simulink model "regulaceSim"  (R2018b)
settings: Solver=ode5  StartTime=0.0  StopTime=80  FixedStep=0.001  RelTol=1e-3  AbsTol=1e-6
undefined symbols (not defined in the file or in its folder): Crane3D_Center
libraries: simulink x5

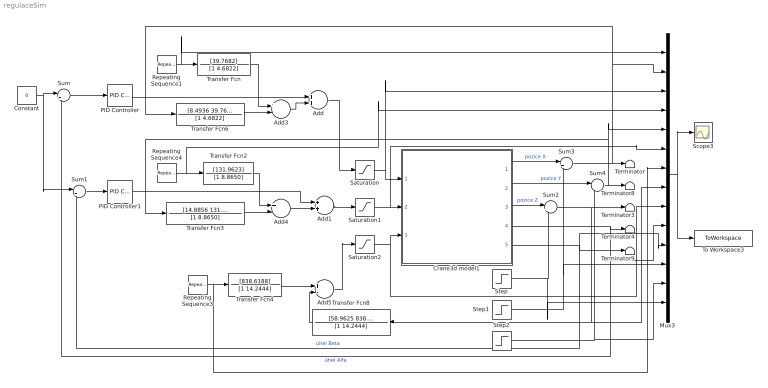
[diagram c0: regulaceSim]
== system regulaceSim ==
  Add : Sum
  Add1 : Sum
  Add3 : Sum  Inputs=+-
  Add4 : Sum  Inputs=+-
  Add5 : Sum  Inputs=+-
  Constant : Constant  Value=0
  Crane3d model1 : Subsystem  mask{RR=off, x0=[0.001, 0, 0.001, 0, 0, 0, 0, 0, 0.001, 0, -1]}
      mask prompts: RR "Model with constant length"; x0 "Initial conditions:[x,x',y,y',alfa,alfa',beta,beta',z,z',t]"
  Mux3 : Mux  Inputs=14
  PID Controller : simulink/Continuous/PID Controller  Controller=P  Form=Parallel  TimeDomain=Continuous-time  SampleTime=-1  IntegratorMethod=Forward Euler  FilterMethod=Forward Euler  ControllerParametersSource=internal  P=-4.5  I=1  D=0  UseFilter=on  N=100  TunerSelectOption=Transfer Function Based (PID Tuner App)  InitialConditionSource=internal  InitialConditionForIntegrator=0  InitialConditionForFilter=0  DifferentiatorICPrevScaledInput=0  ExternalReset=none  TrackingMode=off  Kt=1  LimitOutput=off  UpperSaturationLimit=inf  LowerSaturationLimit=-inf  LinearizeAsGain=on  AntiWindupMode=none  Kb=1  POutMin=[]  POutMax=[]  IOutMin=[]  IOutMax=[]  DOutMin=[]  DOutMax=[]  NOutMin=[]  NOutMax=[]  SumOutMin=[]  SumOutMax=[]  SaturationOutMin=[]  SaturationOutMax=[]  PParamMin=[]  PParamMax=[]  IParamMin=[]  IParamMax=[]  DParamMin=[]  DParamMax=[]  NParamMin=[]  NParamMax=[]  KbParamMin=[]  KbParamMax=[]  KtParamMin=[]  KtParamMax=[]  KbOutMin=[]  KbOutMax=[]  KtOutMin=[]  KtOutMax=[]  IntegratorOutMin=[]  IntegratorOutMax=[]  FilterOutMin=[]  FilterOutMax=[]  SumI1OutMin=[]  SumI1OutMax=[]  SumI2OutMin=[]  SumI2OutMax=[]  SumI3OutMin=[]  SumI3OutMax=[]  SumI4OutMin=[]  SumI4OutMax=[]  SumDOutMin=[]  SumDOutMax=[]  DifferentiatorOutMin=[]  DifferentiatorOutMax=[]  FilterDiffOutCoefMin=[]  FilterDiffOutCoefMax=[]  ReciprocalOutMin=[]  ReciprocalOutMax=[]  SumDenOutMin=[]  SumDenOutMax=[]  SumNumOutMin=[]  SumNumOutMax=[]  DivideOutMin=[]  DivideOutMax=[]  IntegratorContinuousStateAttributes=''  IntegratorStateMustResolveToSignalObject=off  IntegratorRTWStateStorageClass=Auto  FilterContinuousStateAttributes=''  FilterStateMustResolveToSignalObject=off  FilterRTWStateStorageClass=Auto  ParallelPVariant=InternalParameters  IdealPVariant=Disabled  IVariant=Disabled  DVariant=Disabled  IntegratorVariant=Disabled  SatVariant=Disabled  AWVariant=Disabled  PCopyVariant=Disabled  TRVariant=Disabled  FdbkBlocksVariant=Forward  IdealPFdbkVariant=Disabled  SatFdbkVariant=Disabled  DerivativeFilterVariant=Disabled  NVariant=Disabled  NCopyVariant=Disabled_SignalSpec  FilterICVariant=Disabled  IntegratorICVariant=Disabled  ExternalResetVariant=Disabled  TRSumVariant=Passthrough  SumFdbkVariant=Disabled  SumVariant=Passthrough_P
  PID Controller1 : simulink/Continuous/PID Controller  Controller=P  Form=Parallel  TimeDomain=Continuous-time  SampleTime=-1  IntegratorMethod=Forward Euler  FilterMethod=Forward Euler  ControllerParametersSource=internal  P=-4.5  I=1  D=0  UseFilter=on  N=100  TunerSelectOption=Transfer Function Based (PID Tuner App)  InitialConditionSource=internal  InitialConditionForIntegrator=0  InitialConditionForFilter=0  DifferentiatorICPrevScaledInput=0  ExternalReset=none  TrackingMode=off  Kt=1  LimitOutput=off  UpperSaturationLimit=inf  LowerSaturationLimit=-inf  LinearizeAsGain=on  AntiWindupMode=none  Kb=1  POutMin=[]  POutMax=[]  IOutMin=[]  IOutMax=[]  DOutMin=[]  DOutMax=[]  NOutMin=[]  NOutMax=[]  SumOutMin=[]  SumOutMax=[]  SaturationOutMin=[]  SaturationOutMax=[]  PParamMin=[]  PParamMax=[]  IParamMin=[]  IParamMax=[]  DParamMin=[]  DParamMax=[]  NParamMin=[]  NParamMax=[]  KbParamMin=[]  KbParamMax=[]  KtParamMin=[]  KtParamMax=[]  KbOutMin=[]  KbOutMax=[]  KtOutMin=[]  KtOutMax=[]  IntegratorOutMin=[]  IntegratorOutMax=[]  FilterOutMin=[]  FilterOutMax=[]  SumI1OutMin=[]  SumI1OutMax=[]  SumI2OutMin=[]  SumI2OutMax=[]  SumI3OutMin=[]  SumI3OutMax=[]  SumI4OutMin=[]  SumI4OutMax=[]  SumDOutMin=[]  SumDOutMax=[]  DifferentiatorOutMin=[]  DifferentiatorOutMax=[]  FilterDiffOutCoefMin=[]  FilterDiffOutCoefMax=[]  ReciprocalOutMin=[]  ReciprocalOutMax=[]  SumDenOutMin=[]  SumDenOutMax=[]  SumNumOutMin=[]  SumNumOutMax=[]  DivideOutMin=[]  DivideOutMax=[]  IntegratorContinuousStateAttributes=''  IntegratorStateMustResolveToSignalObject=off  IntegratorRTWStateStorageClass=Auto  FilterContinuousStateAttributes=''  FilterStateMustResolveToSignalObject=off  FilterRTWStateStorageClass=Auto  ParallelPVariant=InternalParameters  IdealPVariant=Disabled  IVariant=Disabled  DVariant=Disabled  IntegratorVariant=Disabled  SatVariant=Disabled  AWVariant=Disabled  PCopyVariant=Disabled  TRVariant=Disabled  FdbkBlocksVariant=Forward  IdealPFdbkVariant=Disabled  SatFdbkVariant=Disabled  DerivativeFilterVariant=Disabled  NVariant=Disabled  NCopyVariant=Disabled_SignalSpec  FilterICVariant=Disabled  IntegratorICVariant=Disabled  ExternalResetVariant=Disabled  TRSumVariant=Passthrough  SumFdbkVariant=Disabled  SumVariant=Passthrough_P
  Repeating Sequence1 : simulink/Sources/Repeating Sequence  rep_seq_t=[0 14.99 15 24.99 25 39.99 40 54.99 55 64.99 65 80]  rep_seq_y=[0.001 0.001 0.4 0.4 0.1 0.1 0.3 0.3 0.5 0.5 Crane3D_Center('X') Crane3D_Center('X')]
  Repeating Sequence3 : simulink/Sources/Repeating Sequence  rep_seq_t=[0 4.99 5 19.99 20 34.99 35 49.99 50 64.99 65 80]  rep_seq_y=[0.001 0.001 0.1 0.1 0.2 0.2 0.3 0.3 0.4 0.4 0.5 0.5]
  Repeating Sequence4 : simulink/Sources/Repeating Sequence  rep_seq_t=[0 7.99 8 29.99 30 39.99 40 59.99 60 69.99 70 80]  rep_seq_y=[0.2 0.2 0.1 0.1 0.5 0.5 0.3 0.3 0.4 0.4 Crane3D_Center('Y') Crane3D_Center('Y')]
  Saturation : Saturate  UpperLimit=1  LowerLimit=-1
  Saturation1 : Saturate  UpperLimit=1  LowerLimit=-1
  Saturation2 : Saturate  UpperLimit=1  LowerLimit=-1
  Scope3 : Scope
  Step : Step  Time=12  After=0.1  SampleTime=0
  Step1 : Step  Time=17  After=0.1  SampleTime=0
  Step2 : Step  Time=45  After=0.1  SampleTime=0
  Sum : Sum  Inputs=|+-
  Sum1 : Sum  Inputs=|+-
  Sum2 : Sum  Inputs=|++
  Sum3 : Sum  Inputs=|++
  Sum4 : Sum  Inputs=|++
  Terminator{,3..4,8..9} (5 alike) : Terminator
  To Workspace3 : ToWorkspace  VariableName=CraneRegSim  SaveFormat=Timeseries  SampleTime=-1
  Transfer Fcn : TransferFcn  Numerator=[39.7682]  Denominator=[1 4.6822]
  Transfer Fcn2 : TransferFcn  Numerator=[131.9623]  Denominator=[1 8.8650]
  Transfer Fcn3 : TransferFcn  Numerator=[14.8856 131.9623]  Denominator=[1 8.8650]
  Transfer Fcn4 : TransferFcn  Numerator=[838.6188]  Denominator=[1 14.2444]
  Transfer Fcn6 : TransferFcn  Numerator=[8.4936 39.7682]  Denominator=[1 4.6822]
  Transfer Fcn8 : TransferFcn  Numerator=[58.9625 838.6188]  Denominator=[1 14.2444]
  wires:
  Crane3d model1/3(Z Position) -> Sum2/1  "pozice Z"
  Crane3d model1/4(X Angle) -> Terminator4/1, Mux3/10, Sum/2  "úhel Alfa"
  Saturation/1 -> Mux3/3, Crane3d model1/1(X PWM)
  Saturation1/1 -> Mux3/6, Crane3d model1/2(Y PWM)
  Sum/1 -> PID Controller/1
  Sum1/1 -> PID Controller1/1
  PID Controller1/1 -> Add1/1
  Transfer Fcn4/1 -> Add5/1
  Transfer Fcn3/1 -> Add4/2
  Add1/1 -> Saturation1/1
  Add4/1 -> Add1/2
  Add/1 -> Saturation/1
  Repeating Sequence3/1 -> Mux3/7, Transfer Fcn4/1
  Repeating Sequence1/1 -> Mux3/1, Transfer Fcn/1
  Transfer Fcn2/1 -> Add4/1
  Add5/1 -> Saturation2/1
  Saturation2/1 -> Crane3d model1/3(Z PWM), Mux3/9
  Transfer Fcn6/1 -> Add3/2
  Add3/1 -> Add/2
  Constant/1 -> Sum1/1, Sum/1
  Transfer Fcn8/1 -> Add5/2
  Sum2/1 -> Mux3/8, Transfer Fcn8/1, Terminator3/1
  Mux3/1 -> To Workspace3/1, Scope3/1
  Step/1 -> Mux3/14, Sum2/2
  PID Controller/1 -> Add/1
  Repeating Sequence4/1 -> Mux3/4, Transfer Fcn2/1
  Transfer Fcn/1 -> Add3/1
  Crane3d model1/5(Y Angle) -> Sum1/2, Mux3/11, Terminator9/1  "úhel Beta"
  Crane3d model1/1(X Posiion) -> Sum3/1  "pozice X"
  Step1/1 -> Mux3/12, Sum3/2
  Sum4/1 -> Transfer Fcn3/1, Mux3/5, Terminator8/1
  Crane3d model1/2(Y Position) -> Sum4/1  "pozice Y"
  Step2/1 -> Mux3/13, Sum4/2
  Sum3/1 -> Mux3/2, Transfer Fcn6/1, Terminator/1

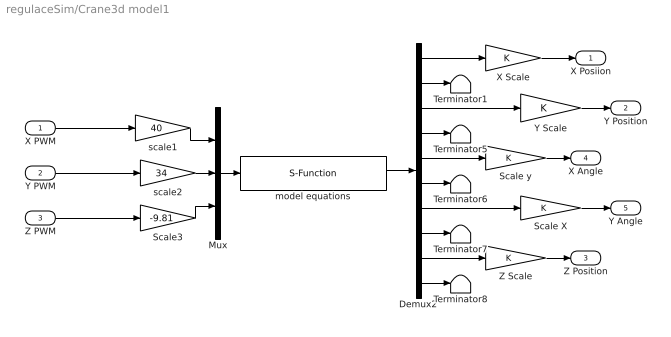
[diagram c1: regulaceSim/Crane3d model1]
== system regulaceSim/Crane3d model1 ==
  X PWM : Inport
  Y PWM : Inport  Port=2
  Z PWM : Inport  Port=3
  Demux2 : Demux  Outputs=10
  Mux : Mux  Inputs=3
  Scale X : Gain
  Scale y : Gain
  Scale3 : Gain  Gain=-9.81
  Terminator{1,5..8} (5 alike) : Terminator
  X Scale : Gain
  Y Scale : Gain
  Z Scale : Gain
  model equations : S-Function  FunctionName=model3dddm  Parameters=x0(1) x0(2) x0(3) x0(4) x0(5) x0(6) x0(7) x0(8) x0(9) x0(10) x0(11) RR  SFunctionDeploymentMode=off  EnableBusSupport=off
  scale1 : Gain  Gain=40
  scale2 : Gain  Gain=34
  X Posiion : Outport  Tag=X Position
  Y Position : Outport  Port=2
  Z Position : Outport  Port=3
  X Angle : Outport  Port=4
  Y Angle : Outport  Port=5
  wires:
  X PWM/1 -> scale1/1
  scale1/1 -> Mux/1
  Z PWM/1 -> Scale3/1
  Scale3/1 -> Mux/3
  Y PWM/1 -> scale2/1
  scale2/1 -> Mux/2
  Demux2/10 -> Terminator8/1
  Demux2/8 -> Terminator7/1
  Demux2/6 -> Terminator6/1
  Demux2/4 -> Terminator5/1
  Demux2/2 -> Terminator1/1
  Demux2/7 -> Scale X/1
  Scale X/1 -> Y Angle/1
  Demux2/5 -> Scale y/1
  Scale y/1 -> X Angle/1
  Demux2/9 -> Z Scale/1
  Z Scale/1 -> Z Position/1
  Demux2/3 -> Y Scale/1
  Demux2/1 -> X Scale/1
  X Scale/1 -> X Posiion/1
  model equations/1 -> Demux2/1
  Y Scale/1 -> Y Position/1
  Mux/1 -> model equations/1
